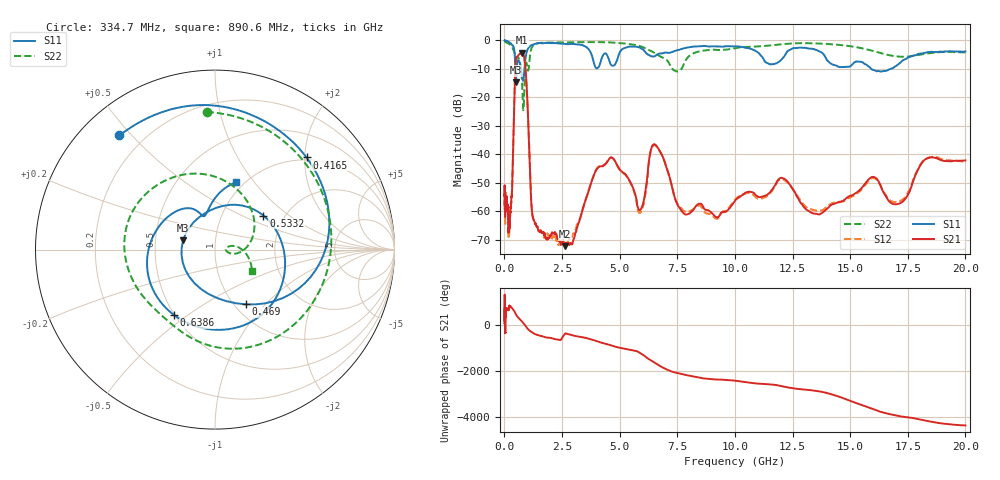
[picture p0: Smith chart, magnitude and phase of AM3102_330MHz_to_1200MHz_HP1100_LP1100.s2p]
! Date/Time: Tue, Sep 11, 2018 5:21 PM
! Network Analyzer: Agilent Technologies E8362B Rev: A.07.50.63
! Sweep from 0.010 to 20.000 GHz, 1601 Points, Sweep Type: LOG
! Power Supply: 4.949 V, 0.001 A
# Hz S DB R 50
!freq MagS11 AngS11 MagS21 AngS21 MagS12 AngS12 MagS22 AngS22
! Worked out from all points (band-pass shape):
!   1601 points, 10 MHz to 20 GHz, reference 50 ohm
!   highest |S21| = -4.34 dB at 765 MHz (marker M1); lowest = -72.2 dB at 2.631 GHz (marker M2)
!   |S21| within 3 dB of the highest: 492.9 MHz to 883.8 MHz (391 MHz wide, 56.8 % of centre)
!   lowest |S11| = -14.7 dB at 496.5 MHz (marker M3), VSWR 1.45, Z = 34.7 + j3.66 ohm
!   |S11| at or under -10 dB: 471.6 MHz to 529.5 MHz (57.94 MHz wide, 11.6 % of centre); 724.6 MHz to 870.3 MHz (145.7 MHz wide, 18.3 % of centre); 15.91 GHz to 16.76 GHz (851.5 MHz wide, 5.21 % of centre)
!   |S22| runs from -24.5 to -0.2 dB; largest |S21 - S12| = 0.0098
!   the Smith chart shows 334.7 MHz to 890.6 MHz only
!   S11 on the Smith chart (normalised r, x): 334.7 MHz: 0.11, +0.46; 416.5 MHz: 0.95, +2.04; 469 MHz: 1.13, -0.78; 533.2 MHz: 1.57, +0.67; 638.6 MHz: 0.50, -0.45; 890.6 MHz: 0.92, +0.81
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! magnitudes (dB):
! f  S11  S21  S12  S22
! 10 MHz  0.0  -54.2  -51.4  -0.2
! 35.55 MHz  -0.1  -58.7  -58.6  -0.5
! 126.4 MHz  -0.3  -58.6  -59.5  -0.9
! 209.1 MHz  -0.7  -65.3  -67.5  -1.2
! 334.7 MHz  -1.6  -52.3  -52.1  -2.3
! 416.5 MHz  -2.8  -25.2  -25.2  -3.9
! 447.2 MHz  -4.6  -15.8  -15.9  -4.6
! 469 MHz  -9.1  -10.7  -10.7  -5.5
! 496.5 MHz  -14.7  -7.0  -7.1  -6.5
! 533.2 MHz  -9.6  -5.8  -5.9  -6.3
! 638.6 MHz  -7.3  -4.9  -5.0  -6.6
! 765 MHz  -12.0  -4.3  -4.4  -14.4
! 890.6 MHz  -8.1  -7.8  -7.9  -12.4
! 1.201 GHz  -1.6  -60.4  -60.5  -2.3
! 1.59 GHz  -1.0  -66.7  -67.2  -0.9
! 2.631 GHz  -1.3  -72.2  -70.8  -0.7
! 4.564 GHz  -7.5  -41.5  -41.3  -0.7
! 5.652 GHz  -2.2  -53.4  -53.7  -1.6
! 6.549 GHz  -5.5  -36.6  -36.8  -4.6
! 7.697 GHz  -3.0  -60.0  -59.1  -9.8
! 9.047 GHz  -2.1  -61.0  -61.6  -3.3
! 20 GHz  -3.9  -42.1  -42.6  -4.2
